FUNCTION_BLOCK TL_NCI_Axis
VAR_INPUT
	TorquePermission	: BOOL;
	Referenced			: BOOL;
	Enable				: BOOL;
	Reset				: BOOL;
	followMe			: BOOL;
	inc_per_unit	: LREAL := 1E7; (* use 10000 inc/deg or 1E7 inc/m *)
END_VAR
VAR_OUTPUT
	messageHandler  : TL_AxisMessageHandler;
END_VAR
VAR
	/// NC > Axis > Drive > Inputs > nState1 
	State1	AT %Q*		: BYTE;
	/// NC > Axis > Drive > Inputs > nState4
	State4	AT %Q*		: BYTE;
	/// NC > Axis > Drive > Outputs > nDataOut1
	PosCmd	AT %I*		: DWORD;
	/// NC > Axis > Enc > Inputs > nDataIn1
	PosAct	AT %Q*		: DWORD;
	
	nciAxis 			: AXIS_REF;

	FB_MC_Power			: MC_Power;
	FB_MC_Reset			: MC_Reset;
	FB_Reset1			: R_TRIG;
	FB_Reset2			: R_TRIG;
	
	twincatEventLib		: TL_TwinCatError;  // Events of the library-axis
	twincatEventDrv		: TL_TwinCatError;  // Events of a drive axis

END_VAR

(* --------------------------------------------- *)
(* Triamec Motion AG, 6340 Baar, Switzerland     *)
(* Sample Code may be adapted to customer need   *)
(* --------------------------------------------- *)

// messageHandler.messageString shows the message string of the drive, valid if messageHandler.done
;

METHOD CallFastPosAct
VAR_INPUT
	iPositionAct		: LREAL;
END_VAR

(* coerse position to DINT range *)
IF ABS(iPositionAct * inc_per_unit) < 16#7FFFFFFF  THEN
	PosAct := DINT_TO_DWORD(LREAL_TO_DINT(iPositionAct * inc_per_unit));
ELSIF iPositionAct < 0 THEN
	PosAct := 16#80000000;
ELSE
	PosAct := 16#7FFFFFFF;
END_IF
END_METHOD

METHOD CallFastPosCmd : LREAL
VAR_INPUT
END_VAR
CallFastPosCmd := DINT_TO_LREAL(DWORD_TO_DINT(PosCmd)) / inc_per_unit;
END_METHOD

METHOD CallSlow
VAR_IN_OUT
	axis				: TL_MC_AXIS_REF;
END_VAR
(*
  Sercos Status Word
  Status1 = 16#4? DriveOn  
  Status1 = 16#8? Feedhold  
  Status1 = 16#C? TorquePermission  
*)
IF NOT Enable THEN
	State1 :=    0;
	State4 :=    4;
ELSIF TorquePermission THEN
	State1 :=16#C8;
	State4 :=    4;
ELSE
	State1 :=16#C0;
	State4 :=    4;
END_IF
IF Referenced THEN
	State1 :=    State1 + 1;
END_IF

(* enable the NCI module *)
FB_MC_Power.Enable			:= Enable;
FB_MC_Power.Enable_Negative	:= TRUE;
FB_MC_Power.Enable_Positive	:= TRUE;
FB_MC_Power.Override		:= 100;
FB_MC_Power(Axis := nciAxis);

FB_Reset1(CLK:=NOT followMe);
FB_Reset2(CLK:=Reset);
FB_MC_Reset.Execute			:= FB_Reset1.Q OR FB_Reset2.Q;
FB_MC_Reset(Axis := nciAxis);

// This reads the drive message string into messageHandler.messageString and then sets messageHandler.done
messageHandler.execute := axis.messageId >= TL_Message.Error; // show only errors
messageHandler(axis:=axis, Trialink:=gTrialink);

// This generates a TwinCAT event in case of an axis library error and an axis drive error
twincatEventLib.Execute	:= gTrialink.Done AND NOT (gTrialink.Error OR axis.simulate);
twincatEventLib.errorId	:= axis.errorId;
twincatEventLib.source	:= TL_EventSourceId.AxisLib; // See source entry in the ecpx file triamecEventsTrialinkLib*.ecpx
twincatEventLib.par1	:= axis.iAxis;
twincatEventLib();

twincatEventDrv.Execute	:= twincatEventLib.Execute AND axis.messageId>=TL_Message.Error; // show only errors 
twincatEventDrv.errorId	:= axis.messageId;
twincatEventDrv.source	:= TL_EventSourceId.AxisDrive; // See source entry in the ecpx file triamecEventsDrive*.ecpx
twincatEventDrv.par1	:= axis.iAxis;
twincatEventDrv();
END_METHOD

END_FUNCTION_BLOCK
